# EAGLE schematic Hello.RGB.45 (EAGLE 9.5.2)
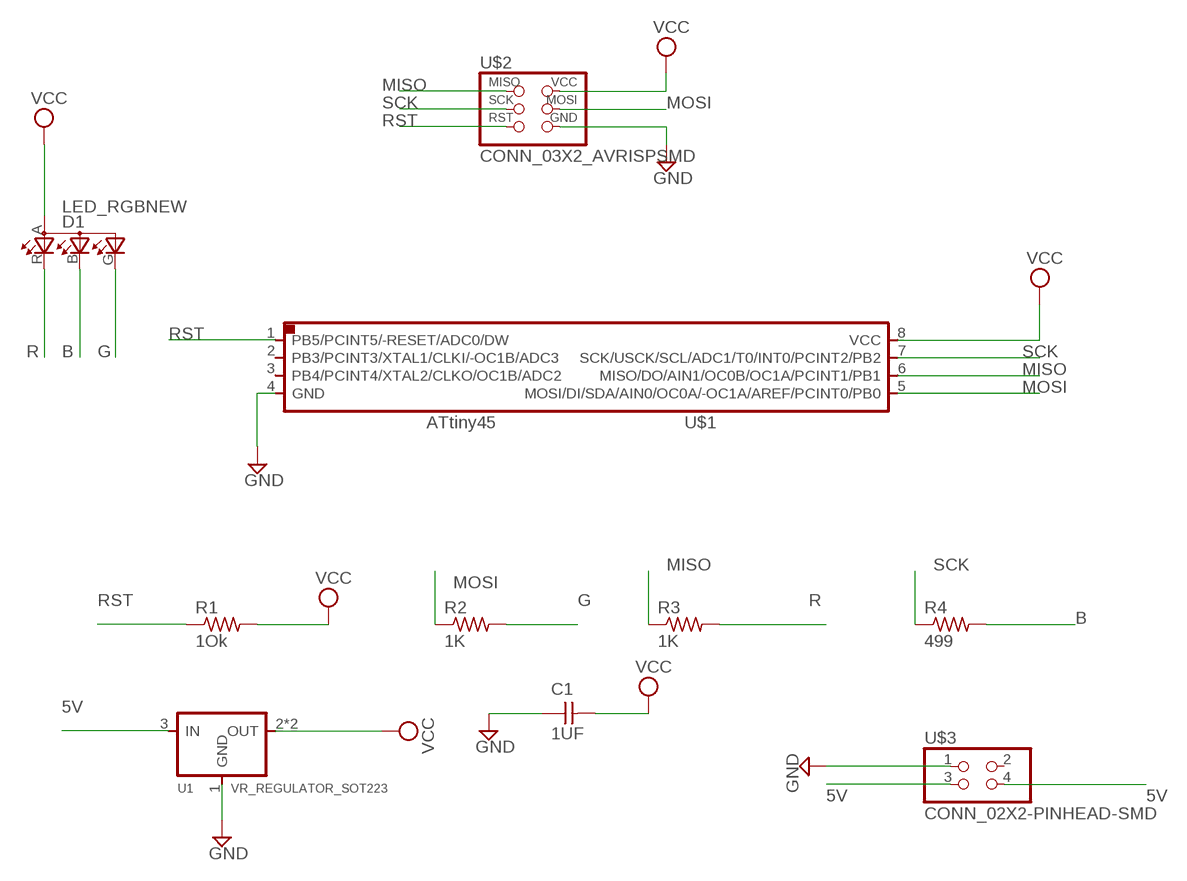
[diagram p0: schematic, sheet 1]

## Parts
C1  1UF  CAP_UNPOLARIZED  [C1206]
D1  LED_RGBNEW  [P-LCC-4]
R1  1Ok  R1206  [R1206]
R2  1K  R1206  [R1206]
R3  1K  R1206  [R1206]
R4  499  R1206  [R1206]
U1  VR_REGULATOR_SOT223  [SOT223]
U$1  UC_ATTINY45SI  [SOIC8]
U$2  CONN_03X2_AVRISPSMD  [2X03SMD]
U$3  CONN_02X2-PINHEAD-SMD  [2X02SMD]

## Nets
5V: U1.3(IN) U$3.3 U$3.4
B: D1.B(CBLUE) R4.2
G: D1.G(CGREEN) R2.2
GND: C1.1 U1.1(GND) U$1.4(GND) U$2.6(GND) U$3.1
MISO: R3.1 U$1.6(MISO/DO/AIN1/OC0B/OC1A/PCINT1/PB1) U$2.1(MISO)
MOSI: R2.1 U$1.5(MOSI/DI/SDA/AIN0/OC0A/-OC1A/AREF/PCINT0/PB0) U$2.4(MOSI)
R: D1.R(CRED) R3.2
RST: R1.1 U$1.1(PB5/PCINT5/-RESET/ADC0/DW) U$2.5(RST)
SCK: R4.1 U$1.7(SCK/USCK/SCL/ADC1/T0/INT0/PCINT2/PB2) U$2.3(SCK)
VCC: C1.2 D1.A(A2) R1.2 U1.2(OUT) U1.4(OUT) U$1.8(VCC) U$2.2(VCC)
Unconnected: U$1.2(PB3/PCINT3/XTAL1/CLKI/-OC1B/ADC3) U$1.3(PB4/PCINT4/XTAL2/CLKO/OC1B/ADC2) U$3.2

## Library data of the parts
C1 = fab:CAP_UNPOLARIZED
D1 = fab:LED_RGBNEW
R1-R4 = fab:R: Resistor (US Symbol)
U1 = fab:VR_REGULATOR_SOT223
U$1 = fab:UC_ATTINY45
U$2 = fab:CONN_03X2_AVRISP
U$3 = fab:CONN_02X2-PINHEAD-SMD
